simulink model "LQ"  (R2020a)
settings: Solver=VariableStepAuto  StartTime=0.0  StopTime=10.0  RelTol=1e-3
PreLoadFcn:
  | initParams
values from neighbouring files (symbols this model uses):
  a = 10    [initParams.m]
  b = 1    [initParams.m]
  K = 10    [initParams.m]
  x0 = [0.2;0.1]    [initParams.m]
  xd = [x1d;0;0]    [initParams.m]

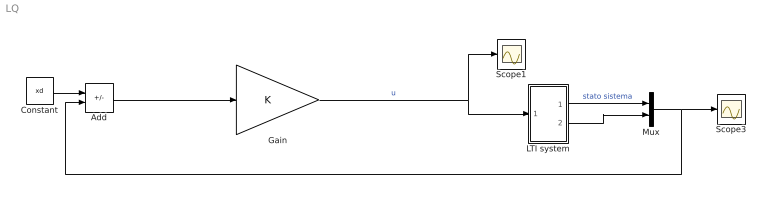
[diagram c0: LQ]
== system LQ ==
  Add : Sum  Inputs=+-
  Constant : Constant  Value=xd
  Gain : Gain  Gain=K  Multiplication=Matrix(K*u) (u vector)
  LTI system : Subsystem
  Mux : Mux  Inputs=2
  Scope1 : Scope
  Scope3 : Scope
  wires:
  Gain/1 -> LTI system/1(u), Scope1/1  "u"
  LTI system/1(x1) -> Mux/1  "stato sistema"
  Mux/1 -> Add/2, Scope3/1
  LTI system/2(x2) -> Mux/2
  Constant/1 -> Add/1
  Add/1 -> Gain/1

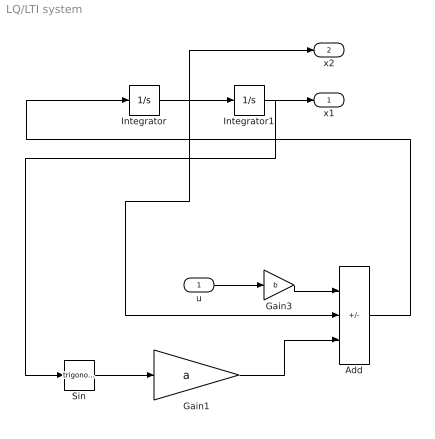
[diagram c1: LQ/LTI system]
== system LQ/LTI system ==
  u : Inport
  Add : Sum  Inputs=+--
  Gain1 : Gain  Gain=a
  Gain3 : Gain  Gain=b
  Integrator : Integrator  InitialCondition=x0(2)
  Integrator1 : Integrator  InitialCondition=x0(1)
  Sin : Trigonometry
  x1 : Outport
  x2 : Outport  Port=2
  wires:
  Add/1 -> Integrator/1
  Gain3/1 -> Add/1
  Gain1/1 -> Add/3
  Sin/1 -> Gain1/1
  u/1 -> Gain3/1
  Integrator1/1 -> Sin/1, x1/1
  Integrator/1 -> Add/2, x2/1, Integrator1/1
